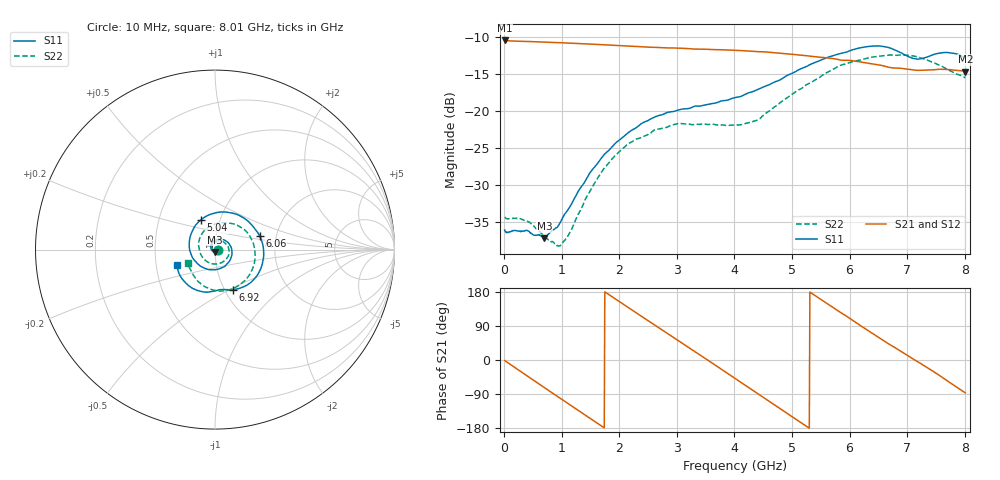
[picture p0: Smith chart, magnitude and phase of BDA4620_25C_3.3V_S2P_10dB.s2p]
!Agilent Technologies,E5071B,MY42404982,A.09.10
!Date: Wed May 06 08:50:32 2026
!Data & Calibration Information:
!Freq	S11:SOLT2(ON)	S21:SOLT2(ON)	S12:SOLT2(ON)	S22:SOLT2(ON)
# Hz S RI R 50
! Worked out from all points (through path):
!   801 points, 10 MHz to 8.01 GHz, reference 50 ohm
!   highest |S21| = -10.43 dB at 10 MHz (marker M1); lowest = -14.6 dB at 8.01 GHz (marker M2)
!   group delay of S21, straight-line fit = 280 ps
!   lowest |S11| = -37.3 dB at 700 MHz (marker M3), VSWR 1.03, Z = 49.8 - j1.35 ohm
!   |S11| at or under -10 dB: start of sweep to end of sweep
!   |S22| runs from -38.3 to -12.4 dB; largest |S21 - S12| = 0.0013
!   S11 on the Smith chart (normalised r, x): 10 MHz: 1.03, -0.00; 5.04 GHz: 0.81, +0.28; 6.06 GHz: 1.64, +0.26; 6.92 GHz: 1.09, -0.52; 8.01 GHz: 0.64, -0.12
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1e7  0.0156 -0.00108  0.3008 -0.00648  0.301 -0.00646  0.019 -0.00112
4.1e8  0.0102 -0.0116  0.2172 -0.2013  0.2172 -0.2017  0.0141 -0.0109
7e8  -0.00204 -0.0135  0.087 -0.2802  0.0869 -0.2805  0.00327 -0.0138
9.8e8  -0.0166 -0.00594  -0.0581 -0.2846  -0.0583 -0.2849  -0.00957 -0.00766
1.35e9  -0.0237 0.0201  -0.2174 -0.186  -0.2176 -0.186  -0.0172 0.0141
1.65e9  -0.00998 0.0445  -0.2779 -0.0492  -0.2783 -0.0491  -0.00826 0.0353
1.94e9  0.0182 0.058  -0.2627 0.0928  -0.2632 0.093  0.014 0.0484
2.32e9  0.0633 0.0462  -0.1448 0.2323  -0.1451 0.2326  0.0503 0.0412
2.68e9  0.093 0.00359  0.0191 0.2688  0.0193 0.2691  0.0743 0.0124
3e9  0.0878 -0.0493  0.158 0.2153  0.1584 0.2154  0.0775 -0.026
3.39e9  0.0405 -0.1002  0.2548 0.0658  0.2552 0.0655  0.045 -0.0676
4.01e9  -0.0852 -0.089  0.1708 -0.1933  0.1709 -0.1937  -0.0505 -0.0629
4.5e9  -0.144 0.0201  -0.0372 -0.2491  -0.0375 -0.2497  -0.0912 0.0205
5.04e9  -0.0781 0.1656  -0.2166 -0.1075  -0.2168 -0.1073  -0.0286 0.1297
5.35e9  0.0217 0.2086  -0.2338 0.0201  -0.234 0.0202  0.0508 0.1492
5.67e9  0.141 0.1874  -0.1814 0.138  -0.1815 0.1383  0.1378 0.128
6.06e9  0.2496 0.0749  -0.052 0.2126  -0.052 0.2131  0.2142 0.0321
6.37e9  0.2671 -0.0645  0.0627 0.2  0.063 0.2002  0.2214 -0.0652
6.68e9  0.1913 -0.1894  0.1465 0.1329  0.147 0.1332  0.1788 -0.1588
6.92e9  0.1004 -0.2232  0.1826 0.0659  0.1831 0.0659  0.1171 -0.2094
7.56e9  -0.0866 -0.2308  0.1452 -0.1253  0.1455 -0.1257  -0.0845 -0.1857
8.01e9  -0.2105 -0.0885  0.0096 -0.1851  0.00971 -0.1856  -0.1504 -0.0743
